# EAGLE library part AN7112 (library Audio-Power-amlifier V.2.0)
0,5 W AUDIO POWER AMPLIFIER
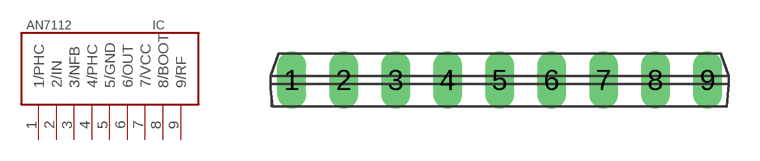
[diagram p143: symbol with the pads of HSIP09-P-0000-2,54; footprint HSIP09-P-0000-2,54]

Designator prefix IC

## AN7112  [HSIP09-P-0000-2,54]
1  1/PHC
2  2/IN  in
3  3/NFB  in
4  4/PHC
5  5/GND  pwr
6  6/OUT  out
7  7/VCC  pwr
8  8/BOOT
9  9/RF

## Footprint HSIP09-P-0000-2,54 (pad centres in mm)
drill 0.9 long: 1 -10.16,0; 2 -7.62,0; 3 -5.08,0; 4 -2.54,0; 5 0,0; 6 2.54,0; 7 5.08,0; 8 7.62,0; 9 10.16,0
